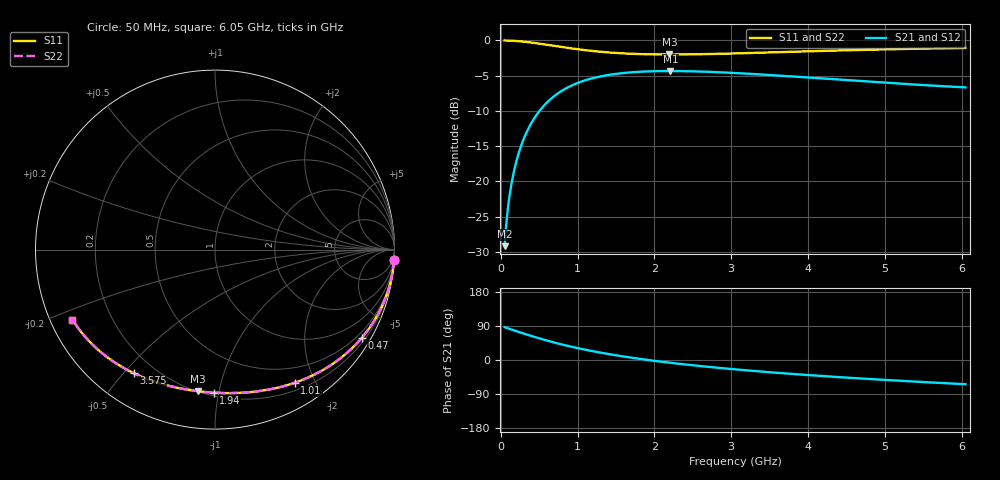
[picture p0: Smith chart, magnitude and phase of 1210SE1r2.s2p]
! AVX Thin Film Operation		Date: August 2001
! Description: Accu-P® Series, Thin Film, SMD, RF Capacitor
! Part Number: 12101J1R2ABT
! 50 MHz  -  6.05 GHz
! Serial Measurements
# mhz S db R 50
!	S11		S21		S12		S22
!	dB	Phase	dB	Phase	dB	Phase	dB	Phase
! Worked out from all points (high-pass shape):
!   401 points, 50 MHz to 6.05 GHz, reference 50 ohm
!   highest |S21| = -4.34 dB at 2.21 GHz (marker M1); lowest = -29.2 dB at 50 MHz (marker M2)
!   |S21| within 3 dB of the highest: 766.5 MHz to end of sweep
!   lowest |S11| = -2.0 dB at 2.195 GHz (marker M3), VSWR 8.74, Z = 10.1 - j43.2 ohm
!   |S11| at or under -10 dB: nowhere
!   |S22| runs from -2.0 to 0.0 dB; largest |S21 - S12| = 0
!   S11 on the Smith chart (normalised r, x): 50 MHz: 0, -33; 470 MHz: 0.32, -3.58; 1.01 GHz: 0.29, -1.73; 1.94 GHz: 0.22, -0.97; 3.575 GHz: 0.12, -0.53; 6.05 GHz: 0.06, -0.23
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50  -0.01 -3.4  -29.17 86.6  -29.17 86.6  -0.01 -3.4
125  -0.03 -8.6  -21.26 81.4  -21.26 81.4  -0.03 -8.6
155  -0.05 -10.6  -19.43 79.4  -19.43 79.4  -0.05 -10.6
200  -0.08 -13.7  -17.27 76.3  -17.27 76.3  -0.08 -13.7
260  -0.14 -17.7  -15.10 72.3  -15.10 72.3  -0.14 -17.7
320  -0.20 -21.6  -13.42 68.4  -13.42 68.4  -0.20 -21.6
470  -0.41 -31.0  -10.50 59.0  -10.50 59.0  -0.41 -31.0
590  -0.59 -38.0  -8.93 52.0  -8.93 52.0  -0.59 -38.0
725  -0.82 -45.4  -7.66 44.6  -7.66 44.6  -0.82 -45.4
1010  -1.26 -59.0  -5.99 31.0  -5.99 31.0  -1.26 -59.0
1055  -1.32 -61.0  -5.81 29.0  -5.81 29.0  -1.32 -61.0
1460  -1.75 -76.3  -4.80 13.7  -4.80 13.7  -1.75 -76.2
1940  -1.97 -90.6  -4.38 -0.6  -4.38 -0.6  -1.97 -90.6
2060  -1.99 -93.7  -4.36 -3.7  -4.36 -3.7  -1.99 -93.7
2195  -2.00 -97.0  -4.34 -7.0  -4.34 -7.0  -2.00 -97.0
2210  -2.00 -97.4  -4.34 -7.4  -4.34 -7.4  -2.00 -97.4
2630  -1.95 -106.6  -4.42 -16.6  -4.42 -16.6  -1.95 -106.6
3050  -1.84 -114.6  -4.62 -24.7  -4.62 -24.7  -1.84 -114.6
3575  -1.68 -123.4  -4.95 -33.4  -4.95 -33.4  -1.68 -123.4
4055  -1.53 -130.5  -5.29 -40.5  -5.29 -40.5  -1.53 -130.5
5060  -1.25 -143.2  -6.03 -53.2  -6.03 -53.2  -1.25 -143.2
6050  -1.06 -153.9  -6.66 -63.9  -6.66 -63.9  -1.06 -153.9
